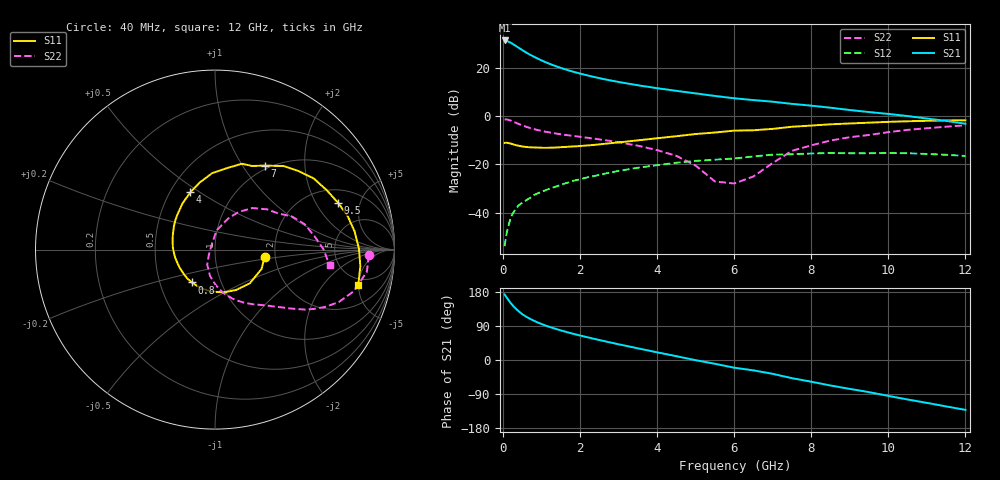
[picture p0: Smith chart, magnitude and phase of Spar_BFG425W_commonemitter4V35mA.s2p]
! Filename: 435bfg425.001
! BFG425W Field C1
! V1=8.387E-001V,V2=4.000E+000V, I1=4.655E-004A, I2=3.500E-002A
# GHz  S  MA  R 50
!  S11  S21  S12  S22
!Freq(GHz)  Mag  Ang  Mag  Ang  Mag  Ang  Mag  Ang
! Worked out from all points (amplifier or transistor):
!   44 points, 40 MHz to 12 GHz, reference 50 ohm
!   highest |S21| = 31.4 dB at 40 MHz (marker M1)
!   |S21| within 3 dB of that: start of sweep to 401.3 MHz
!   unconditionally stable (mu >= 1): start of sweep to 96.68 MHz; 938.2 MHz to end of sweep
!   at 700 MHz: K = 0.94, MSG = 29.8 dB, |S12| = -34.0 dB
!   at 2.4 GHz: K = 1.21, MAG = 17.6 dB, |S12| = -24.7 dB
!   at 12 GHz: K = 1.38, MAG = 3.0 dB, |S12| = -16.5 dB
!   S11 on the Smith chart (normalised r, x): 40 MHz: 1.75, -0.16; 800 MHz: 0.73, -0.28; 4 GHz: 0.63, +0.46; 7 GHz: 0.95, +1.27; 9.5 GHz: 2.75, +3.12; 12 GHz: 4.14, -4.96
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0.04  0.279 -8.7  37.31 173.0  0.002 45.3  0.858 -2.1
0.1  0.281 -22.4  36.37 163.9  0.004 63.3  0.855 -8.3
0.2  0.27 -43.9  33.45 149.8  0.008 65.9  0.808 -16.6
0.3  0.254 -62.1  29.84 138.5  0.011 65.9  0.749 -23.0
0.4  0.243 -78.5  26.46 129.0  0.014 64.8  0.691 -27.6
0.5  0.235 -93.4  23.5 120.8  0.016 63.4  0.643 -30.9
0.6  0.229 -105.2  21 114.3  0.018 62.6  0.602 -33.7
0.8  0.224 -125.2  17.15 103.6  0.023 61.5  0.539 -37.6
1  0.221 -141.0  14.35 94.9  0.027 60.7  0.494 -40.7
1.3  0.222 -159.5  11.43 84.2  0.033 59.0  0.446 -45.0
1.7  0.232 -178.7  8.94 72.4  0.042 56.2  0.4 -50.4
2.2  0.247 162.3  6.983 59.7  0.054 51.3  0.355 -57.9
3  0.285 137.9  5.128 41.5  0.073 41.8  0.288 -70.8
4  0.348 113.2  3.808 20.2  0.096 27.9  0.197 -89.0
4.5  0.384 102.7  3.353 10.0  0.108 20.3  0.15 -100.6
5.5  0.458 81.9  2.627 -10.1  0.125 4.8  0.044 -140.3
6.5  0.51 66.0  2.158 -27.4  0.146 -7.5  0.056 98.9
7  0.545 59.2  1.996 -36.5  0.159 -15.2  0.107 85.4
8.5  0.678 35.8  1.498 -67.3  0.172 -44.2  0.312 47.9
9.5  0.733 21.0  1.217 -84.9  0.17 -60.7  0.407 29.6
10.5  0.784 7.5  1.006 -104.2  0.17 -79.2  0.519 15.8
12  0.822 -13.7  0.697 -131.6  0.149 -108.9  0.645 -7.9
